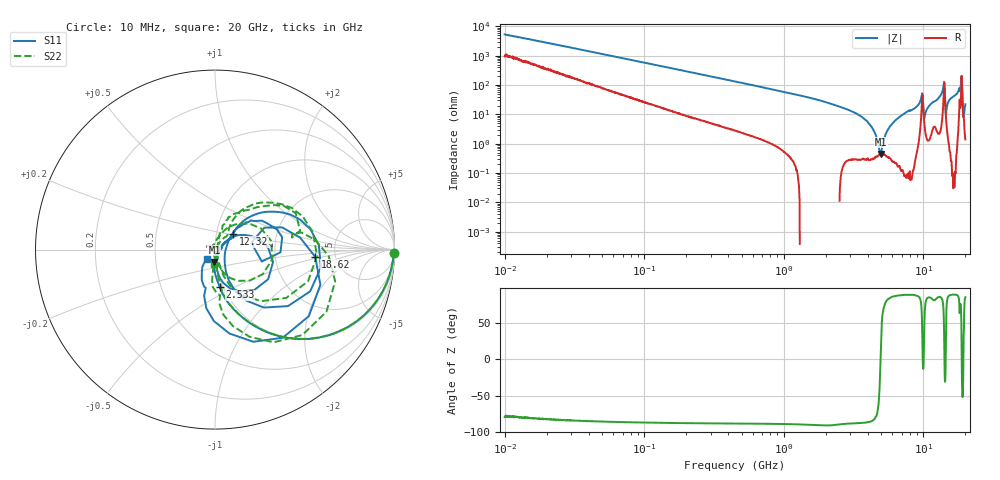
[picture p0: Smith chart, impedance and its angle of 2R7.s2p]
!Keysight Technologies,P5008B,MY61100088,A.16.20.02
!Date: Monday, October 30, 2023 16:31:01
!Correction: S11(C  2-Port  )
!S21(C  2-Port  )
!S12(C  2-Port  )
!S22(C  2-Port  )
!S2P File: Measurements: S11, S21, S12, S22:Log Frequency Sweep
# Hz S  dB  R 50
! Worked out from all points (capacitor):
!   1601 points, 10 MHz to 20 GHz, reference 50 ohm
!   read as one part in series: C = 2.96 pF near 10.39 MHz
!   lowest |Z| = 447 mohm at 4.948 GHz (marker M1)
!   series resonance near 4.934 GHz, so ESL is about 350 pH
!   S11 on the Smith chart (normalised r, x): 10 MHz: open; 2.533 GHz: 0.96, -0.42; 12.32 GHz: 1.20, +0.21; 18.62 GHz: 3.49, -0.41; 20 GHz: 0.91, -0.09
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1e7  -0.03 -1.1  -34.57 78.7  -34.57 78.6  -0.03 -1.1
3.555162e7  -0.06 -3.6  -24.17 81.6  -24.17 81.5  -0.06 -3.6
1.263918e8  -0.27 -12.2  -13.62 75.5  -13.63 75.6  -0.27 -12.2
4.472136e8  -2.02 -37.0  -4.54 51.9  -4.55 51.9  -2.02 -36.9
1.589917e9  -9.08 -72.4  -0.54 18.4  -0.55 18.4  -9.08 -72.2
2.532576e9  -13.51 -82.7  -0.21 8.4  -0.21 8.4  -13.67 -81.1
4.948411e9  -23.23 -92.4  -0.04 -4.0  -0.04 -4.0  -23.25 -85.1
5.652411e9  -26.28 -90.0  -0.02 -6.6  -0.02 -6.6  -26.44 -90.3
6.867879e9  -32.47 -49.5  0.00 -10.9  0.00 -10.9  -34.23 -142.9
7.697294e9  -29.22 5.4  0.00 -13.9  -0.00 -13.9  -30.30 142.3
8.344716e9  -32.70 -1.1  0.01 -16.3  0.00 -16.4  -34.13 135.2
8.918577e9  -28.06 30.1  -0.02 -19.2  -0.02 -19.3  -28.89 91.2
9.807503e9  -9.61 -12.1  -3.03 -26.6  -3.03 -26.7  -10.00 9.0
1.083639e10  -31.56 -9.4  -0.07 -20.5  -0.08 -20.5  -40.29 14.0
1.231939e10  -17.53 41.0  -0.31 -26.9  -0.31 -27.0  -17.74 54.3
1.380717e10  -6.68 24.9  -2.04 -45.1  -2.04 -45.2  -6.93 34.2
1.454787e10  -17.38 -63.4  -0.56 -15.2  -0.56 -15.2  -20.01 -73.4
1.511139e10  -20.56 34.7  -0.11 -26.8  -0.11 -26.9  -20.55 72.9
1.577149e10  -15.62 44.1  -0.15 -32.5  -0.16 -32.6  -15.22 69.1
1.742604e10  -11.54 37.2  -0.49 -45.4  -0.49 -45.5  -11.00 51.1
1.862442e10  -5.03 -4.2  -5.27 -65.2  -5.28 -65.3  -3.96 -3.1
2e10  -23.47 -131.1  -0.17 -30.8  -0.18 -30.8  -21.99 -92.4
